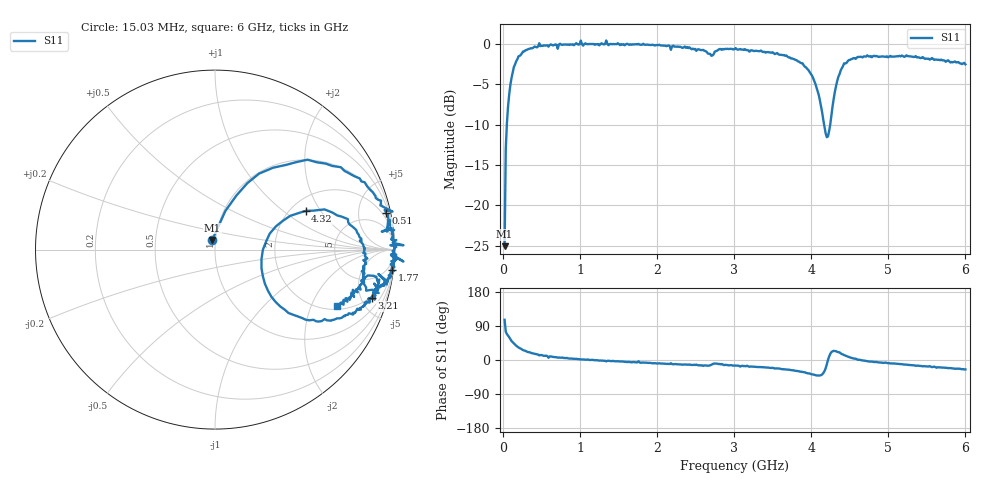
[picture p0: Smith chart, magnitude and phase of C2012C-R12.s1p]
!	Network	Analyzer	HP8753E.07.74:	Oct	30	2002	Serial	No.	JP38451487
!	Hewlett-Packard
!	7	Sep	2009	12:14:06
!	Frequency	S11
#	HZ	S	RI	R	50
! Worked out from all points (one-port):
!   400 points, 15.03 MHz to 6 GHz, reference 50 ohm
!   lowest |S11| = -25.1 dB at 15.03 MHz (marker M1), VSWR 1.12, Z = 48.2 + j5.18 ohm
!   |S11| at or under -10 dB: start of sweep to 44.1 MHz; 4.165 GHz to 4.244 GHz (79.31 MHz wide, 1.89 % of centre)
!   S11 on the Smith chart (normalised r, x): 15.03 MHz: 0.96, +0.10; 510 MHz: 1.21, +9.33; 1.77 GHz: 1, -17; 3.21 GHz: 1.87, -6.05; 4.32 GHz: 2.39, +1.48; 6 GHz: 2.18, -3.11
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1.502992e7  -0.0154 0.0536
3.002985e7  0.0576 0.215
6.00297e7  0.18 0.37
1.050295e8  0.396 0.472
2.550287e8  0.807 0.396
4.650277e8  0.989 0.212
5.100274e8  0.952 0.203
5.850271e8  0.958 0.1
7.650262e8  0.98 0.112
1.005025e9  1.05 0.0244
1.035025e9  0.977 0.0245
1.335023e9  1.05 -0.0663
1.515022e9  0.982 -0.0649
1.770021e9  0.985 -0.114
2.265019e9  0.947 -0.188
2.595017e9  0.886 -0.246
2.700016e9  0.825 -0.183
2.805016e9  0.915 -0.167
3.015015e9  0.912 -0.242
3.210014e9  0.872 -0.27
3.765011e9  0.719 -0.369
4.05001e9  0.438 -0.364
4.200009e9  0.259 -0.0533
4.320008e9  0.505 0.216
4.425008e9  0.74 0.17
4.515007e9  0.8 0.0841
5.265004e9  0.819 -0.188
6e9  0.679 -0.314
